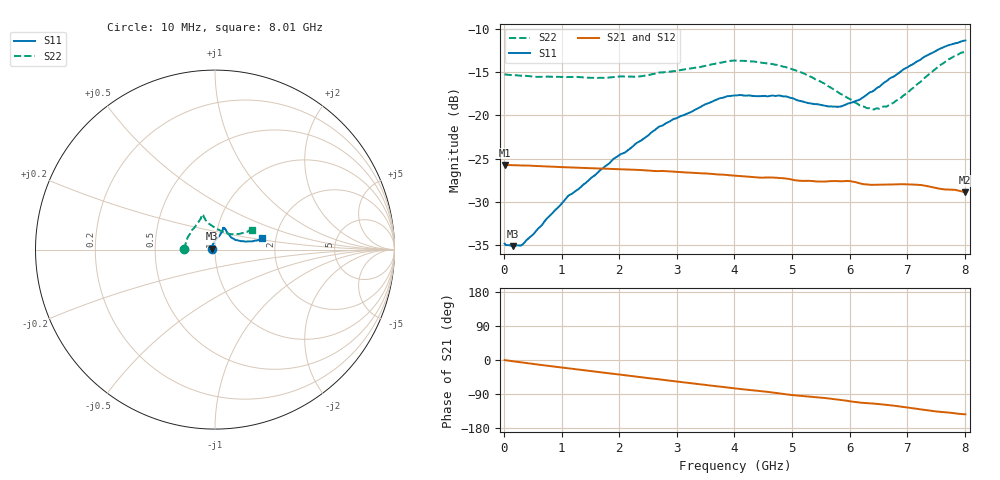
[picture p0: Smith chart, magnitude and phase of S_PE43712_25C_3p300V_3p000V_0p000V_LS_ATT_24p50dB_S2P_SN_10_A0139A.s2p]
! DEVICE ID: PE43712
! File Path: z:\PE43713\PE43713_CHAR_NOM_04292014\AMB\3p300\LS_ATT_24p50dB\PE43713_AMB_3p300V_3p000V_0p000V_LS_ATT_24p50dB_S2P_SN_10_A0139A.s2p
! Serial: 10
! Lot: A0139A
! Temp: 25C
! VDD: 3.300
! VSS: 0.000
! Control_Hi: 3.000
! Control_Lo: 0.000
! Attenuation Step: 24.50dB
! Port 1: RF1
! Port 2: RF2
! ThroughPath:1-2
! IDD: 0.0001450328
! ISS: -1.37e-007
#  Hz  S  RI  R  50
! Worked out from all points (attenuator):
!   801 points, 10 MHz to 8.01 GHz, reference 50 ohm
!   highest |S21| = -25.75 dB at 20 MHz (marker M1); lowest = -28.9 dB at 8 GHz (marker M2)
!   lowest |S11| = -35.2 dB at 160 MHz (marker M3), VSWR 1.04, Z = 48.4 + j0.524 ohm
!   |S11| at or under -10 dB: start of sweep to end of sweep
!   |S22| runs from -19.3 to -12.7 dB; largest |S21 - S12| = 0.0002
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1e7  -0.0181 0.000662  0.0516 -0.000246  0.0516 -0.000202  -0.1726 0.00117
2e7  -0.0179 0.00121  0.0516 -0.000421  0.0516 -0.000413  -0.1724 0.00204
1.6e8  -0.0166 0.00541  0.0514 -0.00305  0.0514 -0.00304  -0.1705 0.0111
3.3e8  -0.0151 0.00972  0.0508 -0.00615  0.0508 -0.00609  -0.1681 0.0202
1.1e9  -0.0101 0.0322  0.0464 -0.0185  0.0465 -0.0186  -0.1544 0.0625
1.35e9  -0.00647 0.0384  0.0445 -0.0221  0.0445 -0.0221  -0.1484 0.074
1.91e9  0.00507 0.056  0.0392 -0.0292  0.0392 -0.0292  -0.1301 0.1045
2.35e9  0.0169 0.0684  0.0342 -0.0341  0.0342 -0.0341  -0.1127 0.1245
2.68e9  0.0272 0.081  0.0301 -0.0368  0.0301 -0.0368  -0.0994 0.1458
3.71e9  0.0448 0.1157  0.0158 -0.0426  0.0158 -0.0426  -0.0754 0.1853
4.01e9  0.0473 0.1215  0.0116 -0.0433  0.0117 -0.0432  -0.0751 0.1934
4.76e9  0.0543 0.1183  0.00167 -0.0434  0.0017 -0.0434  -0.0626 0.185
5.35e9  0.0687 0.0944  -0.0053 -0.0413  -0.00529 -0.0413  -0.0489 0.1586
5.87e9  0.091 0.0671  -0.0114 -0.0399  -0.0113 -0.0399  -0.0142 0.131
6.17e9  0.1095 0.0559  -0.0154 -0.0374  -0.0153 -0.0374  0.0136 0.1136
6.38e9  0.1264 0.052  -0.0165 -0.036  -0.0164 -0.036  0.0366 0.1024
6.68e9  0.155 0.0464  -0.0193 -0.0347  -0.0192 -0.0347  0.0717 0.0893
7.2e9  0.2022 0.0462  -0.0252 -0.0305  -0.0252 -0.0304  0.1264 0.087
7.55e9  0.2356 0.0518  -0.0273 -0.0259  -0.0272 -0.0259  0.1667 0.0961
7.81e9  0.2537 0.0579  -0.0285 -0.0236  -0.0284 -0.0237  0.1925 0.1057
8e9  0.2633 0.0626  -0.0288 -0.0215  -0.0287 -0.0216  0.2043 0.1098
8.01e9  0.2638 0.0632  -0.0288 -0.0215  -0.0287 -0.0216  0.2049 0.1098
